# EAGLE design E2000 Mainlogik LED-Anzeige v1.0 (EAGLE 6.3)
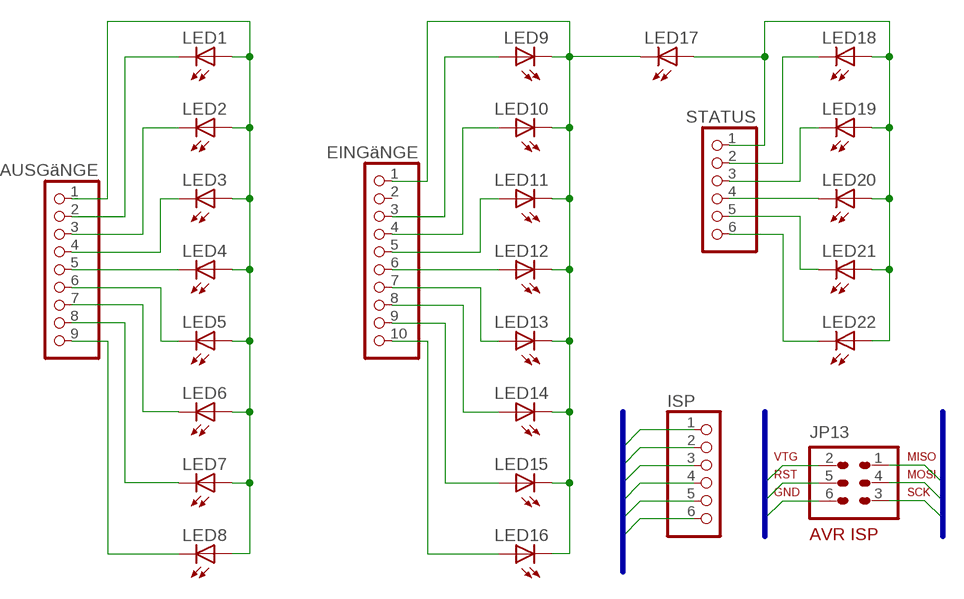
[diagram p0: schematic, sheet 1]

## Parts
AUSGäNGE  PINHD-1X9  [1X09]
EINGäNGE  PINHD-1X10  [1X10]
ISP  PINHD-1X6  [1X06]
JP13  AVR-ISP-6  [AVR-ISP-6]
LED1  LED3MM  [LED3MM]
LED2  LED3MM  [LED3MM]
LED3  LED3MM  [LED3MM]
LED4  LED3MM  [LED3MM]
LED5  LED3MM  [LED3MM]
LED6  LED3MM  [LED3MM]
LED7  LED3MM  [LED3MM]
LED8  LED3MM  [LED3MM]
LED9  LED3MM  [LED3MM]
LED10  LED3MM  [LED3MM]
LED11  LED3MM  [LED3MM]
LED12  LED3MM  [LED3MM]
LED13  LED3MM  [LED3MM]
LED14  LED3MM  [LED3MM]
LED15  LED3MM  [LED3MM]
LED16  LED3MM  [LED3MM]
LED17  LED3MM  [LED3MM]
LED18  LED3MM  [LED3MM]
LED19  LED3MM  [LED3MM]
LED20  LED3MM  [LED3MM]
LED21  LED3MM  [LED3MM]
LED22  LED3MM  [LED3MM]
STATUS  PINHD-1X6  [1X06]

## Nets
+12V: AUSGäNGE.1 LED1.A LED2.A LED3.A LED4.A LED5.A LED6.A LED7.A LED8.A
GND: EINGäNGE.1 ISP.6 JP13.6 LED9.K(C) LED10.K(C) LED11.K(C) LED12.K(C) LED13.K(C) LED14.K(C) LED15.K(C) LED16.K(C) LED17.K(C)
MISO: ISP.1 JP13.1
MOSI: ISP.4 JP13.4
N$2: EINGäNGE.3 LED9.A
N$3: EINGäNGE.4 LED10.A
N$4: EINGäNGE.10 LED16.A
N$5: EINGäNGE.9 LED15.A
N$6: EINGäNGE.8 LED14.A
N$7: EINGäNGE.5 LED11.A
N$8: EINGäNGE.7 LED13.A
N$9: EINGäNGE.6 LED12.A
N$10: AUSGäNGE.2 LED1.K(C)
N$11: AUSGäNGE.3 LED2.K(C)
N$12: AUSGäNGE.4 LED3.K(C)
N$13: AUSGäNGE.5 LED4.K(C)
N$14: AUSGäNGE.9 LED8.K(C)
N$15: AUSGäNGE.8 LED7.K(C)
N$16: AUSGäNGE.7 LED6.K(C)
N$17: AUSGäNGE.6 LED5.K(C)
N$19: LED20.K(C) STATUS.4
N$20: LED18.K(C) STATUS.2
N$21: LED22.K(C) STATUS.6
N$22: LED21.K(C) STATUS.5
N$23: LED19.K(C) STATUS.3
RST: ISP.5 JP13.5
SCK: ISP.3 JP13.3
VCC: LED17.A LED18.A LED19.A LED20.A LED21.A LED22.A STATUS.1
VTG: ISP.2 JP13.2
Unconnected: EINGäNGE.2

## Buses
MISO,MOSI,SCK,VTG,RST,GND

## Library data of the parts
AUSGäNGE = pinhead:PINHD-1X9: PIN HEADER
EINGäNGE = pinhead:PINHD-1X10: PIN HEADER
ISP STATUS = pinhead:PINHD-1X6: PIN HEADER
JP13 = avr-6:AVR-ISP-6: AVR ISP-6 Serial Programming Header
LED1-LED22 = led:LED: LED

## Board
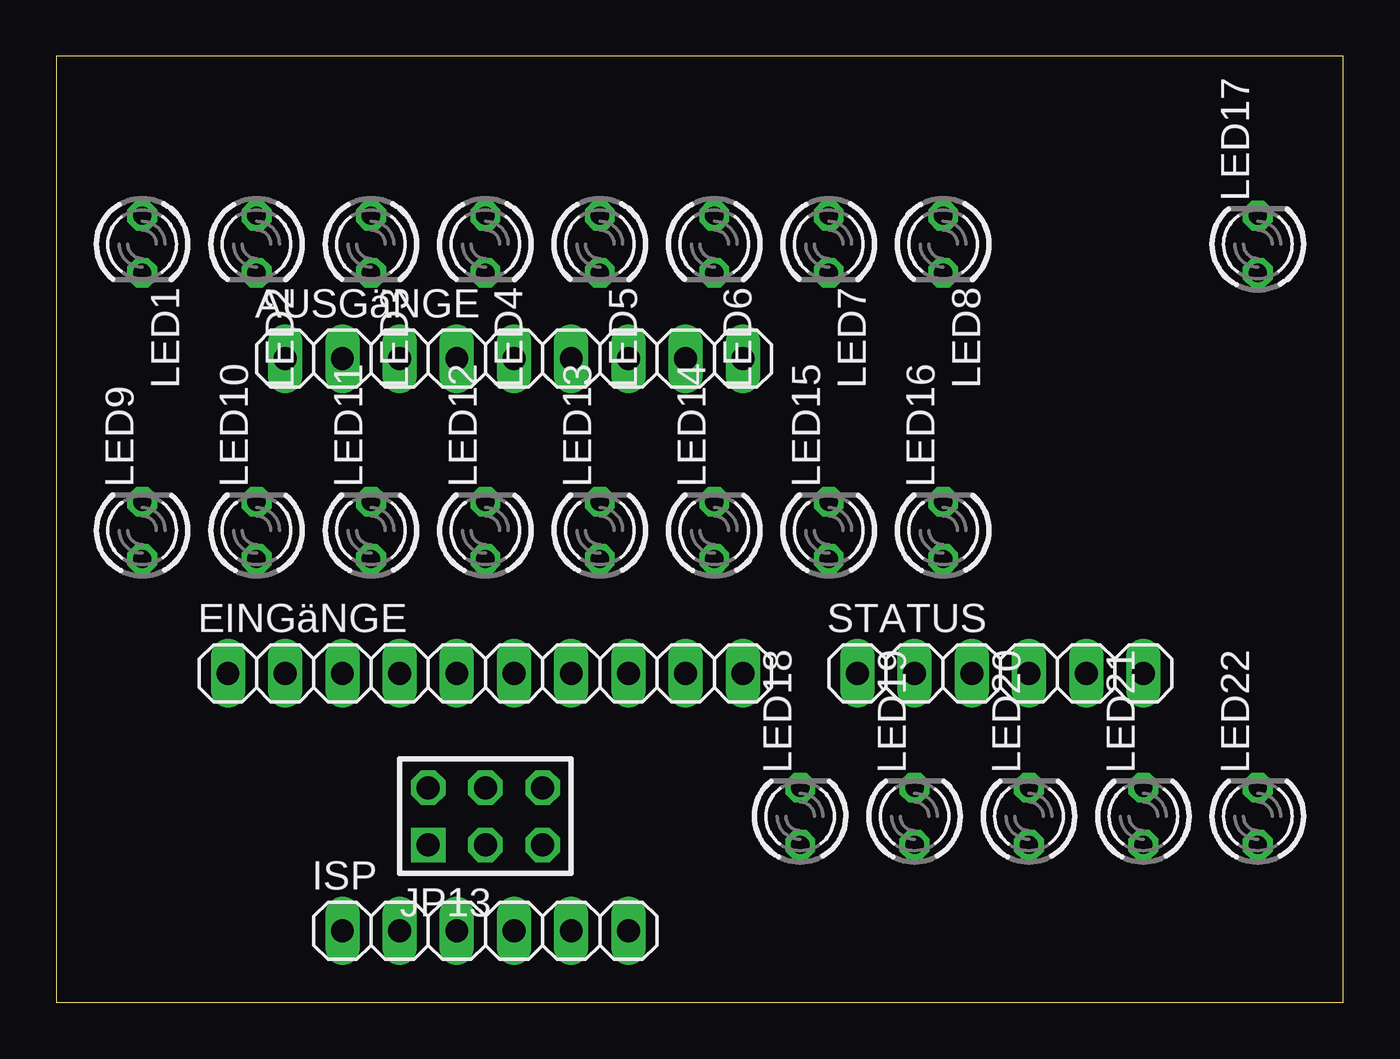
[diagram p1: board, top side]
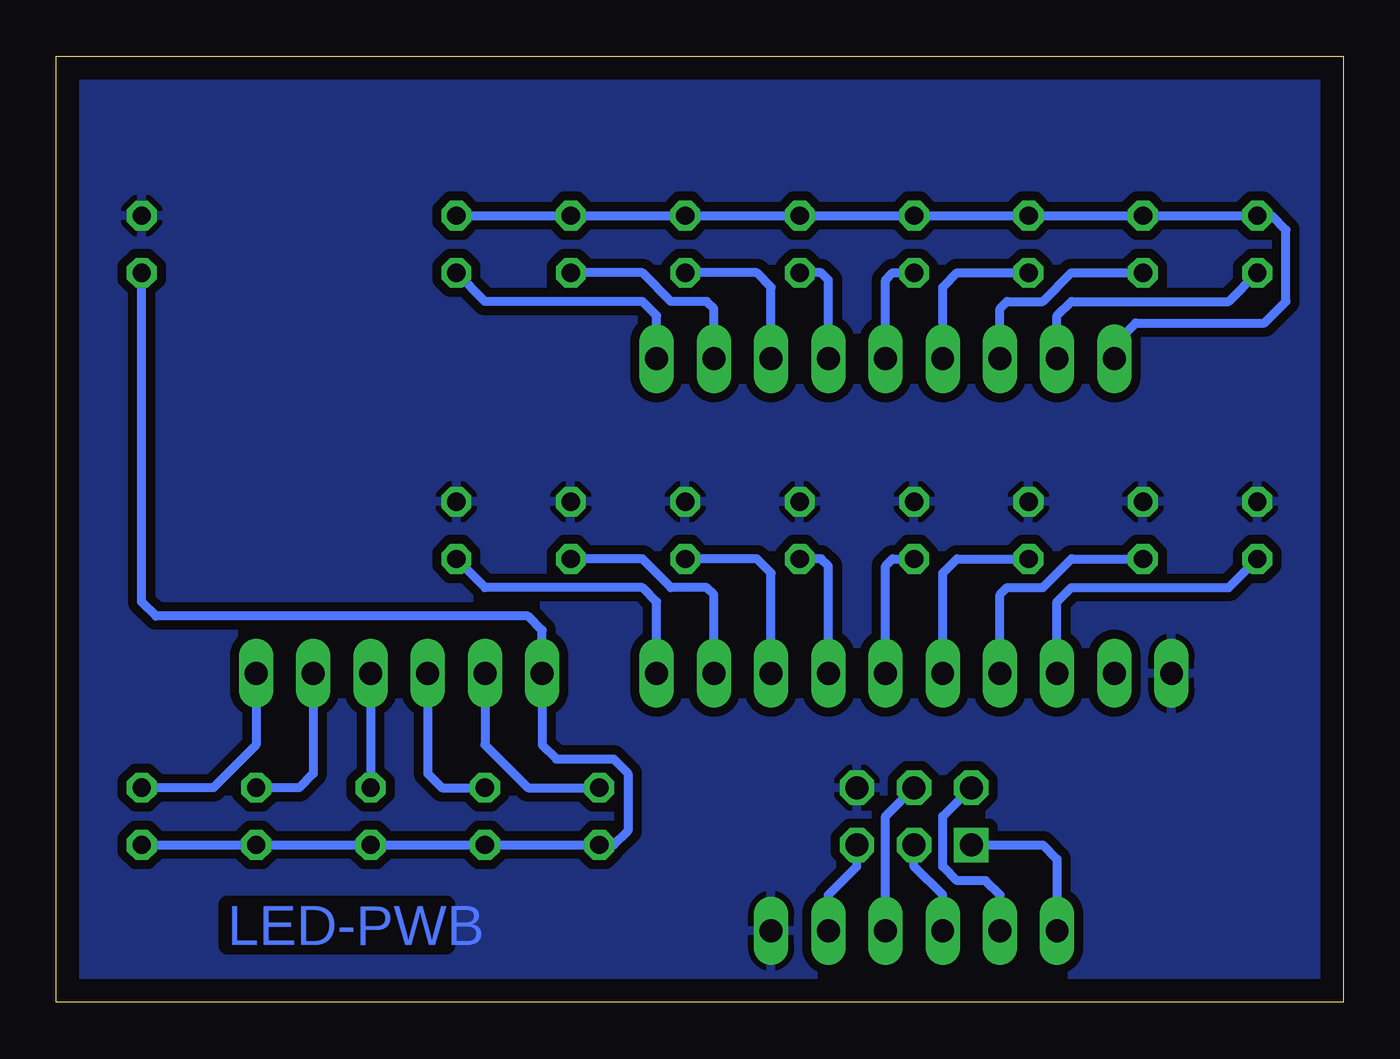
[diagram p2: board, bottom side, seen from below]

Size 57.13 x 42 mm. Coordinates in mm from the lower left corner, seen from the top.
Outline: 0,0 57.13,0 57.13,42 0,42 0,0
Copper layers (1*16): Top 0.035mm / dielectric 1.5mm / Bottom 0.035mm
Design rules "default": minimum track width 10mil, minimum drill 24mil, track to track 8mil, track to pad 8mil, pad to pad 8mil, via to via 8mil, smd to smd 8mil, copper to edge 40mil, drill to drill 8mil, minimum pad ring 10mil, minimum via ring 8mil, stop-mask expansion 4mil, vias tented up to drill 0mil, thermal gap 10mil

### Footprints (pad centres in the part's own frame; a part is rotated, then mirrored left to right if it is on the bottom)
1X09 = drill 1.016 long: 1 -10.16,0; 2 -7.62,0; 3 -5.08,0; 4 -2.54,0; 5 0,0; 6 2.54,0; 7 5.08,0; 8 7.62,0; 9 10.16,0
1X10 = drill 1.016 long: 1 -11.43,0; 2 -8.89,0; 3 -6.35,0; 4 -3.81,0; 5 -1.27,0; 6 1.27,0; 7 3.81,0; 8 6.35,0; 9 8.89,0; 10 11.43,0
1X06 = drill 1.016 long: 1 -6.35,0; 2 -3.81,0; 3 -1.27,0; 4 1.27,0; 5 3.81,0; 6 6.35,0
AVR-ISP-6 = drill 1.016 square: 1 -2.54,-1.27 | drill 1.016 octagon: 2 -2.54,1.27; 3 0,-1.27; 4 0,1.27; 5 2.54,-1.27; 6 2.54,1.27
LED3MM = drill 0.813 octagon: A -1.27,0; K 1.27,0

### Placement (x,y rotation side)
AUSGäNGE  20.32,28.57 0 top
EINGäNGE  19.05,14.61 0 top
ISP  19.05,3.17 0 top
JP13  19.05,8.26 0 top
LED1  3.81,33.66 270 top
LED2  8.89,33.66 270 top
LED3  13.97,33.66 270 top
LED4  19.05,33.66 270 top
LED5  24.13,33.66 270 top
LED6  29.21,33.66 270 top
LED7  34.29,33.66 270 top
LED8  39.37,33.66 270 top
LED9  3.81,20.95 90 top
LED10  8.89,20.95 90 top
LED11  13.97,20.95 90 top
LED12  19.05,20.95 90 top
LED13  24.13,20.95 90 top
LED14  29.21,20.95 90 top
LED15  34.29,20.95 90 top
LED16  39.37,20.95 90 top
LED17  53.34,33.66 90 top
LED18  33.02,8.26 90 top
LED19  38.1,8.26 90 top
LED20  43.18,8.26 90 top
LED21  48.26,8.26 90 top
LED22  53.34,8.26 90 top
STATUS  41.91,14.61 0 top

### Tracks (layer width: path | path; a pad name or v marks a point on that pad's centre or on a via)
+12V
  Bottom 0.406: AUSGäNGE.1 10.16,29.21 9.21,30.16 3.49,30.16 2.54,31.11 2.54,34.29 3.17,34.92 LED1.A LED2.A LED3.A LED4.A LED5.A LED6.A LED7.A LED8.A
GND
  pour Bottom (isolate 0.406): -1.27,43.18 58.42,43.18 58.42,-1.27 -1.27,-1.27
MISO
  Bottom 0.406: JP13.1 13.34,6.99 12.7,6.35 ISP.1
MOSI
  Bottom 0.406: ISP.4 20.32,8.26 JP13.4
N$2
  Bottom 0.406: EINGäNGE.3 12.7,17.78 12.06,18.41 5.08,18.41 LED9.A
N$3
  Bottom 0.406: EINGäNGE.4 15.24,18.1 14.92,18.41 13.34,18.41 12.06,19.68 LED10.A
N$4
  Bottom 0.406: EINGäNGE.10 30.48,17.78 31.11,18.41 38.1,18.41 LED16.A
N$5
  Bottom 0.406: EINGäNGE.9 27.94,18.1 28.26,18.41 29.84,18.41 31.11,19.68 LED15.A
N$6
  Bottom 0.406: EINGäNGE.8 25.4,19.05 26.04,19.68 LED14.A
N$7
  Bottom 0.406: EINGäNGE.5 17.78,19.05 17.14,19.68 LED11.A
N$8
  Bottom 0.406: EINGäNGE.7 22.86,19.37 23.18,19.68 LED13.A
N$9
  Bottom 0.406: EINGäNGE.6 20.32,19.37 20,19.68 LED12.A
N$10
  Bottom 0.406: AUSGäNGE.2 12.7,30.48 12.06,31.11 5.08,31.11 LED1.K
N$11
  Bottom 0.406: AUSGäNGE.3 15.24,30.8 14.92,31.11 13.34,31.11 12.06,32.38 LED2.K
N$12
  Bottom 0.406: AUSGäNGE.4 17.78,31.75 17.14,32.38 LED3.K
N$13
  Bottom 0.406: AUSGäNGE.5 20.32,32.07 20,32.38 LED4.K
N$14
  Bottom 0.406: AUSGäNGE.9 30.48,30.48 31.11,31.11 38.1,31.11 LED8.K
N$15
  Bottom 0.406: AUSGäNGE.8 27.94,30.8 28.26,31.11 29.84,31.11 31.11,32.38 LED7.K
N$16
  Bottom 0.406: AUSGäNGE.7 25.4,31.75 26.04,32.38 LED6.K
N$17
  Bottom 0.406: AUSGäNGE.6 22.86,32.07 23.18,32.38 LED5.K
N$19
  Bottom 0.406: STATUS.4 LED20.K
N$20
  Bottom 0.406: STATUS.2 38.1,11.43 36.2,9.53 LED18.K
N$21
  Bottom 0.406: STATUS.6 48.26,11.43 50.16,9.53 LED22.K
N$22
  Bottom 0.406: STATUS.5 45.72,10.16 46.35,9.53 LED21.K
N$23
  Bottom 0.406: STATUS.3 40.64,10.16 40.01,9.53 LED19.K
RST
  Bottom 0.406: ISP.5 22.86,4.76 21.59,6.03 JP13.5
SCK
  Bottom 0.406: ISP.3 17.78,4.76 19.05,6.03 JP13.3
VCC
  Bottom 0.406: LED22.A LED21.A LED20.A LED19.A LED18.A 32.38,6.99 31.75,7.62 31.75,10.16 32.38,10.79 34.92,10.79 35.56,11.43 STATUS.1 35.56,16.51 36.2,17.14 52.7,17.14 53.34,17.78 LED17.A
VTG
  Bottom 0.406: ISP.2 15.24,4.76 15.88,5.4 17.14,5.4 17.78,6.03 17.78,8.26 JP13.2

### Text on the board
Bottom: LED-PWB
